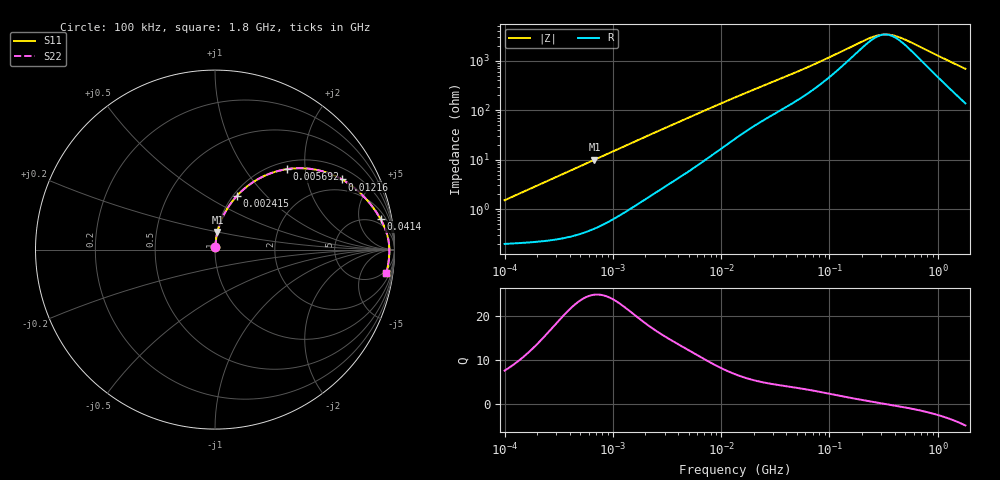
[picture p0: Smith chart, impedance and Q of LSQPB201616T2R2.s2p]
! LSQPB201616T2R2  S-PARAMETER MODEL  ( General Type )
! Model Generated by TAIYO YUDEN Corporation (http://www.ty-top.com)
! Version 2.0
! TAIYO YUDEN Control No. 100810NC14SB-FKC
! Copyright(c) 2008 TAIYO YUDEN CO.,LTD. All Rights Reserved.
! Product Description (link to TY-COMPAS)
! https://ds.yuden.co.jp/TYCOMPAS/or/detail?pn=LSQPB201616T2R2M&u=M
! Products Name : Inductors
! Characteristics :
!  Inductance : 2.2 uH , SRF(min) : 250 MHz , DC Resistance(max) : 0.234 Ohm
!  Rated Current : Saturation :910 mA , Temp Rise : 760 mA (40 degC)
!  Case Size : 2.0 x 1.6 / 0.079 x 0.063 [mm/inch] , Thickness : 1.6 / 0.063 [mm/inch]
!  (Conditions: Temperature = 25 degC , DC Bias Current/Voltage = 0A / 0V)
! External Node Assignments :
!  1  o---GGG---o  2
! GND o---------o GND
! Frequency Range : 0.1MHz  -  1800MHz  [ 402 STEP ]
# MHz S RI R 50
! Freq[MHz].  S11 Real  S11 Imag  S21 Real  S21 Imag  S12 Real  S12 Imag  S22 Real  S22 Imag
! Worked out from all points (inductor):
!   401 points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, 100 kHz to 1.8 GHz, reference 50 ohm
!   read as one part in series: L = 2.37 uH near 105 kHz
!   highest Q = 24.9 at 675.7 kHz (marker M1), where L = 2.35 uH
!   self-resonance near 326.9 MHz
!   S11 on the Smith chart (normalised r, x): 100 kHz: 1.00, +0.03; 2.415 MHz: 1.04, +0.70; 5.692 MHz: 1.14, +1.60; 12.16 MHz: 1.45, +3.28; 41.4 MHz: 3, +10; 1.8 GHz: 4, -14
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0.1  0.00219 0.0149  0.9978 -0.0149  0.9978 -0.0149  0.00219 0.0149
0.253659  0.0037 0.0375  0.9963 -0.0375  0.9963 -0.0375  0.0037 0.0375
0.516129  0.00895 0.0755  0.9911 -0.0755  0.9911 -0.0755  0.00895 0.0755
0.675738  0.0138 0.0982  0.9862 -0.0982  0.9862 -0.0982  0.0138 0.0982
1.409041  0.0494 0.1945  0.9506 -0.1945  0.9506 -0.1945  0.0494 0.1945
2.415258  0.1229 0.3002  0.8771 -0.3002  0.8771 -0.3002  0.1229 0.3002
2.66389  0.1437 0.3214  0.8563 -0.3214  0.8563 -0.3214  0.1437 0.3214
3.846706  0.2473 0.3969  0.7527 -0.3969  0.7527 -0.3969  0.2473 0.3969
5.692459  0.4005 0.4483  0.5995 -0.4483  0.5995 -0.4483  0.4005 0.4483
8.02111  0.5499 0.4472  0.4501 -0.4472  0.4501 -0.4472  0.5499 0.4472
12.1642  0.7076 0.3908  0.2924 -0.3908  0.2924 -0.3908  0.7076 0.3908
13.41641  0.7377 0.3724  0.2623 -0.3724  0.2623 -0.3724  0.7377 0.3724
22.44079  0.8515 0.271  0.1485 -0.271  0.1485 -0.271  0.8515 0.271
41.39926  0.9222 0.1703  0.0778 -0.1703  0.0778 -0.1703  0.9222 0.1703
69.24595  0.9515 0.107  0.0485 -0.107  0.0485 -0.107  0.9515 0.107
235.6695  0.9708 0.0167  0.0292 -0.0167  0.0292 -0.0167  0.9708 0.0167
293.7968  0.9714 0.00537  0.0286 -0.00537  0.0286 -0.00537  0.9714 0.00537
357.3983  0.9716 -0.00451  0.0284 0.00451  0.0284 0.00451  0.9716 -0.00451
413.9822  0.9715 -0.012  0.0285 0.012  0.0285 0.012  0.9715 -0.012
503.6016  0.9713 -0.0225  0.0287 0.0225  0.0287 0.0225  0.9713 -0.0225
999.899  0.9671 -0.0685  0.0329 0.0685  0.0329 0.0685  0.9671 -0.0685
1800  0.9537 -0.1318  0.0463 0.1318  0.0463 0.1318  0.9537 -0.1318
